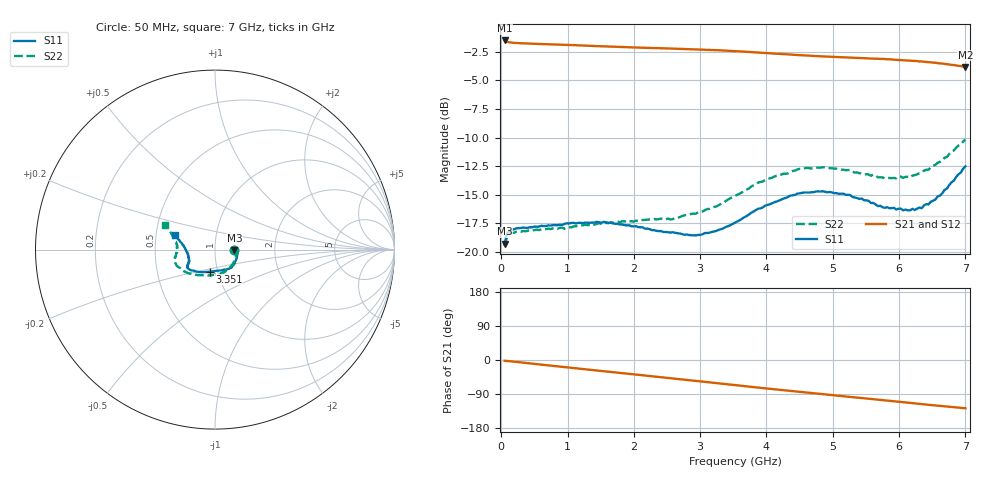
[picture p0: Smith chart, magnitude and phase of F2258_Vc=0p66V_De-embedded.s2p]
! Integrated Device Technology
! Corporate Headquarters
! 6024 Silver Creek Valley Road
! San Jose, CA 95138  USA
! Phone:  1-408-284-8200
! Toll Free:  1-800-223-1366
! Webpage:  http://www.idt.com/
! Timing and RF Division
! 515 Groton Road, Suite 102
! Westford, MA 01886-6024
! Device:  F2258
! Description: Voltage Variable RF Attenuator
! Frequency:  50.0 -  6000.00 MHz
! Package:  3x3 mm Thin QFN Plastic Package: 16 pin
! Ports:  2 RF, 2 DC
!  Pin  1  = NC
!  Pin  2  = NC
!  Pin  3  = RF2  = Port 2
!  Pin  4  = GND
!  Pin  5  = Vdd
!  Pin  6  = NC
!  Pin  7  = VCTRL
!  Pin  8  = NC
!  Pin  9  = GND
!  Pin 10  = RF1  = Port 1
!  Pin 11  = NC
!  Pin 12  = NC
!  Pin 13  = NC
!  Pin 14  = NC
!  Pin 15  = NC
!  Pin 16  = NC
! Vcntrl:  0.660 Volts
! Vdd:  +3.300 Volts
! Current:  1.115 mA
! Data:  The device was measured on a the F2258 evaluation board which has
!  individual transmission lines to the RF pins.  Data was collected
!  using a calibrated network analyzer.  The evaluation board was
!  de-embedded using a TRL calibration technique.
!  The reference plane is the edge of the package pin.
! Misc:  SN 10
!  Action Tracker AT0285
! Date Measured:  2014-12-10
! Date:  2016-01-13  MJV
! Note:
!  Integrated Device Technology supplies this data as a sample of measured
!  data at the package pin for this product.  Your particular data for this
!  product may vary.
!  Data was taken at 25 degrees C.
!  Integrated Device Technology reserves the right to change this data at anytime.
!Freq_(GHz)  S11M_(dB)  S11P_(deg)  S21M_(dB)  S21P_(deg)  S12M_(dB)  S12P_(deg)  S22M_(dB)  S22P_(deg)
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# GHz S dB R 50
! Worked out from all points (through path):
!   201 points, 50 MHz to 7 GHz, reference 50 ohm
!   highest |S21| = -1.50 dB at 50 MHz (marker M1); lowest = -3.8 dB at 7 GHz (marker M2)
!   group delay of S21, straight-line fit = 50.5 ps
!   lowest |S11| = -19.3 dB at 50 MHz (marker M3), VSWR 1.24, Z = 62.2 - j0.5 ohm
!   |S11| at or under -10 dB: start of sweep to end of sweep
!   |S22| runs from -19.5 to -10.2 dB; largest |S21 - S12| = 0.00099
!   S11 on the Smith chart (normalised r, x): 50 MHz: 1.24, -0.01; 3.351 GHz: 0.91, -0.23; 7 GHz: 0.63, +0.11
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0.05  -19.29 -2.1  -1.50 -2.0  -1.50 -2.0  -19.52 -2.7
0.08475  -18.46 -3.5  -1.61 -2.5  -1.61 -2.5  -18.70 -4.1
0.15425  -18.07 -5.6  -1.68 -3.7  -1.69 -3.7  -18.36 -7.2
0.71025  -17.70 -24.4  -1.83 -14.2  -1.83 -14.2  -17.98 -30.5
1.2315  -17.50 -40.9  -1.94 -23.9  -1.94 -23.9  -17.69 -51.7
1.54425  -17.39 -47.9  -2.02 -29.6  -2.01 -29.6  -17.51 -61.7
2.37825  -18.20 -65.5  -2.18 -44.8  -2.17 -44.8  -17.14 -84.2
2.58675  -18.30 -71.5  -2.21 -48.7  -2.20 -48.6  -17.15 -90.8
2.93425  -18.58 -84.7  -2.27 -55.1  -2.28 -55.1  -16.67 -103.2
3.35125  -17.95 -103.7  -2.37 -63.0  -2.38 -63.0  -15.70 -119.9
3.525  -17.47 -111.5  -2.43 -66.3  -2.43 -66.3  -15.13 -126.8
4.0115  -15.90 -130.3  -2.61 -75.3  -2.61 -75.3  -13.62 -143.6
4.46325  -14.92 -141.3  -2.77 -83.5  -2.78 -83.5  -12.80 -155.6
4.7065  -14.79 -144.7  -2.85 -87.8  -2.85 -87.8  -12.70 -160.3
5.2625  -15.04 -150.5  -3.01 -97.4  -3.01 -97.4  -12.85 -169.2
5.6795  -16.01 -155.1  -3.10 -104.5  -3.10 -104.5  -13.49 -175.4
5.85325  -16.20 -159.1  -3.15 -107.7  -3.15 -107.7  -13.54 179.8
6.166  -16.38 -167.2  -3.26 -113.2  -3.26 -113.2  -13.50 173.3
6.2355  -16.35 -170.8  -3.29 -114.4  -3.29 -114.4  -13.29 171.2
6.444  -15.86 -179.3  -3.39 -118.1  -3.39 -118.1  -12.83 166.4
6.722  -14.47 168.7  -3.57 -123.0  -3.56 -123.0  -11.70 159.0
7  -12.53 160.0  -3.82 -127.4  -3.81 -127.4  -10.17 153.6
